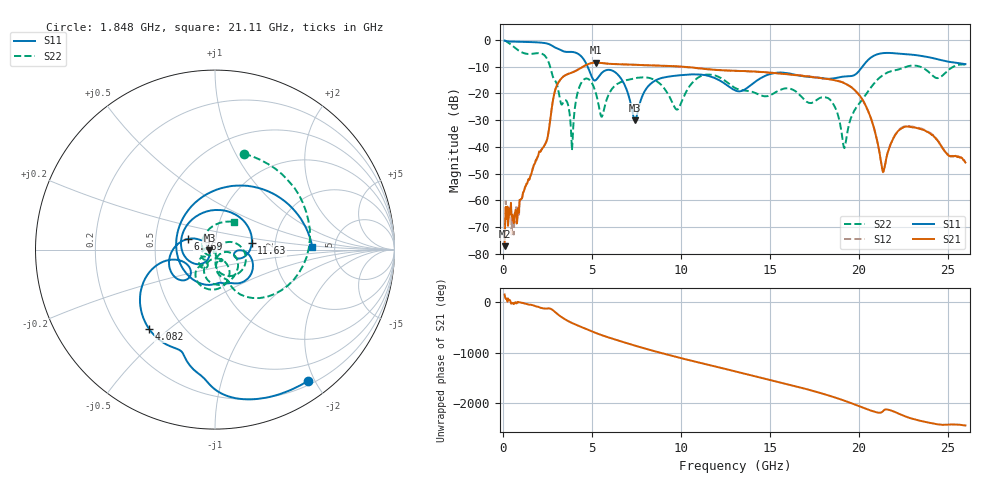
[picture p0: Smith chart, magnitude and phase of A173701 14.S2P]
!  2-Port S-parameters saved by WinCal
! VAR MeasName=S-Parameters (CALIBRATED_DATA) read from VNA (N5245A)
! VAR MeasDate=2017-6-7 10:29:18
! VAR NAME=A173701 14
! VAR FILENAME=A173701 14.S2P
! VAR DATE=2017-6-7 10:29:18
! VAR PHYS_PORTS=1,2
# Hz S DB R 50
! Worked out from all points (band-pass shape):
!   801 points, 100 MHz to 26 GHz, reference 50 ohm
!   highest |S21| = -8.55 dB at 5.248 GHz (marker M1); lowest = -77.1 dB at 100 MHz (marker M2)
!   |S21| within 3 dB of the highest: 4.127 GHz to 12.77 GHz (8.648 GHz wide, 102 % of centre); 12.8 GHz to 12.88 GHz (72.25 MHz wide, 0.563 % of centre)
!   lowest |S11| = -30.1 dB at 7.417 GHz (marker M3), VSWR 1.06, Z = 47 - j0.411 ohm
!   |S11| at or under -10 dB: 4.763 GHz to 20.22 GHz (15.45 GHz wide, 124 % of centre)
!   |S22| runs from -41.2 to -0.3 dB; largest |S21 - S12| = 0.0044
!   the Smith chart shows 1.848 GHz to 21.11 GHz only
!   S11 on the Smith chart (normalised r, x): 1.848 GHz: 0.26, -1.90; 4.082 GHz: 0.32, -0.43; 6.769 GHz: 0.73, +0.09; 11.63 GHz: 1.51, +0.12; 21.11 GHz: 3.36, +0.14
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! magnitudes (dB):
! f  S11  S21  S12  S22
! 100 MHz  -0.3  -77.1  -72.9  -0.3
! 1.848 GHz  -1.0  -45.0  -45.1  -5.1
! 3.046 GHz  -3.2  -16.9  -16.9  -16.8
! 3.856 GHz  -4.5  -12.4  -12.3  -36.7
! 4.082 GHz  -4.8  -11.7  -11.6  -23.9
! 4.438 GHz  -6.4  -10.3  -10.3  -15.8
! 5.248 GHz  -15.0  -8.6  -8.5  -20.4
! 5.571 GHz  -12.3  -8.7  -8.7  -28.7
! 6.769 GHz  -15.8  -9.2  -9.2  -15.5
! 7.417 GHz  -30.1  -9.3  -9.3  -14.4
! 8.744 GHz  -14.7  -9.7  -9.7  -15.9
! 9.812 GHz  -13.4  -9.9  -10.0  -26.1
! 11.63 GHz  -13.6  -11.1  -11.1  -13.0
! 13.05 GHz  -18.9  -11.6  -11.6  -18.0
! 17.39 GHz  -13.9  -13.9  -13.8  -23.5
! 18.46 GHz  -14.5  -14.9  -14.8  -22.9
! 19.2 GHz  -13.7  -16.2  -16.2  -40.5
! 21.11 GHz  -5.3  -40.0  -39.9  -14.6
! 21.37 GHz  -5.0  -49.4  -49.5  -13.2
! 21.69 GHz  -4.9  -40.9  -40.8  -12.0
! 22.96 GHz  -5.6  -32.6  -32.3  -9.7
! 26 GHz  -9.1  -45.8  -45.6  -9.3
